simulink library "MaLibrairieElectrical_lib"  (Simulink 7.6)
settings: Solver=ode45  StartTime=0.0  StopTime=10.0  RelTol=1e-3
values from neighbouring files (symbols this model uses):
  A = [1+j -(1-j);1 -2/(1-j)]    [systeme_AX_B_phaseurs.m]
  K = 0.0005    [parametres.m]
undefined symbols (not defined in the file or in its folder): capa_reelle, F, gcbh, gen_sin_amorti, H, i, MaLibrairieElectrical, nesl_callback, Ohm, op_amp_reel, R_NL, R_NL2, rad, s, thermistance, V, v

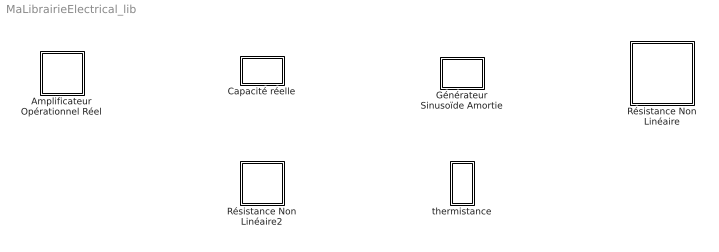
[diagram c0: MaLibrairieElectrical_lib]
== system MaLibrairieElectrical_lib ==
  Amplificateur Opérationnel Réel : Subsystem  DialogController=NetworkEngine.DynNeDlgSource  LoadFcn=nesl_callback('LoadFcn',gcbh);  mask(Amplificateur
Opérationnel Réel){ComponentPath=MaLibrairieElectrical.op_amp_reel, ClassName=op_amp_reel, SchemaVersion=1, A=1e+6, A_unit=1, Re=1e+6, Re_unit=Ohm, Rs=100, Rs_unit=Ohm, Vsat=15, Vsat_unit=V, ie_Log=off, eps_Log=off, is_Log=off, vs_Log=off, LocalVarNames=\, LocalVarDescs=ie\, LocalVarLogging=eps\}
      mask prompts: A "Gain de l'Aop en boucle ouverte"; Re "Résistance d'entrée"; Rs "Résistance de sortie"; Vsat "Tension d'alimentation"
      mask help: Dans cet amplificateur, on tient compte de: - sa résistance d'entrée Re, - sa résistance de sortie Rs, - gain en boucle ouverte, - de la saturation de la sortie à +/-Vsat
      mask init:
      | nesl_preinitmask (gcb);
  Capacité réelle : Subsystem  DialogController=NetworkEngine.DynNeDlgSource  LoadFcn=nesl_callback('LoadFcn',gcbh);  mask(Capacité réelle){ComponentPath=MaLibrairieElectrical.capa_reelle, ClassName=capa_reelle, SchemaVersion=1, C=1e-6, C_unit=F, v0=0, v0_unit=V, Rs=1e-6, Rs_unit=Ohm, Rp=1e+6, Rp_unit=Ohm, Ls=0, Ls_unit=H, vc_Log=off, v_Log=off, i_Log=off, LocalVarNames=\, LocalVarDescs=vc\, LocalVarLogging=v\}
      mask prompts: C "Capacité"; v0 "charge initiale de la capacité"; Rs "Résistance série Rs"; Rp "Résistance parallèle Rp"; Ls "Inductance série Ls"
      mask help: Cette capacité est composée d'une capacité idéale en parallèle à une résistance Rp le tout en série à une résistance Rs et une inductance Ls
      mask init:
      | nesl_preinitmask (gcb);
  Générateur Sinusoïde Amortie : Subsystem  DialogController=NetworkEngine.DynNeDlgSource  LoadFcn=nesl_callback('LoadFcn',gcbh);  mask(Générateur Sinusoïde
Amortie){ComponentPath=MaLibrairieElectrical.gen_sin_amorti, ClassName=gen_sin_amorti, SchemaVersion=1, biais=0, biais_unit=1, w=6.2832, w_unit=1/s, Amp=1, Amp_unit=1, phi=6.2832, phi_unit=rad, a=5, a_unit=1, LocalVarNames=, LocalVarDescs=, LocalVarLogging=[]}
      mask prompts: w "pulsation"; Amp "Amplitude"; phi "Phase"; a "décrément"
      mask help: Ce bloc génère le signal suivant x(t)=Amp exp(-at) sin (wt+phi)+ biais
      mask init:
      | nesl_preinitmask (gcb);
  Résistance Non Linéaire : Subsystem  DialogController=NetworkEngine.DynNeDlgSource  LoadFcn=nesl_callback('LoadFcn',gcbh);  mask(Résistance Non
Linéaire){ComponentPath=MaLibrairieElectrical.R_NL, ClassName=R_NL, SchemaVersion=1, K=10, K_unit=V/A^2, v_Log=off, i_Log=off, LocalVarNames=\, LocalVarDescs=v\, LocalVarLogging=i}
      mask prompts: K "Coefficient de la Résistance non linéaire"
      mask help: Ce composant définit une résistance non linéaire La valeur de la résistance dépend du courant qui la traverse La caractéristique est donnée par la relation entre le courant qui traverse la résistance et la tension à ses bornes U=K*i^2
      mask init:
      | nesl_preinitmask (gcb);
  Résistance Non Linéaire2 : Subsystem  DialogController=NetworkEngine.DynNeDlgSource  LoadFcn=nesl_callback('LoadFcn',gcbh);  mask(Résistance Non
Linéaire2){ComponentPath=MaLibrairieElectrical.R_NL2, ClassName=R_NL2, SchemaVersion=1, R0=10, R0_unit=Ohm, K=10, K_unit=V/A^2, i_Log=off, v_Log=off, LocalVarNames=\, LocalVarDescs=i\, LocalVarLogging=v}
      mask prompts: K "Coefficient de la Résistance non linéaire"
      mask help: Ce composant définit une résistance non linéaire La valeur de la résistance dépend du courant qui la traverse La caractéristique est donnée par la relation entre le courant qui traverse la résistance et la tension à ses bornes U=K*i^2
      mask init:
      | nesl_preinitmask (gcb);
  thermistance : Subsystem  DialogController=NetworkEngine.DynNeDlgSource  LoadFcn=nesl_callback('LoadFcn',gcbh);  mask(thermistance){ComponentPath=MaLibrairieElectrical.thermistance, ClassName=thermistance, SchemaVersion=1, T0=300, T0_unit=K, B=2.9e+3, B_unit=K, R0=100, R0_unit=Ohm, LocalVarNames=, LocalVarDescs=, LocalVarLogging=[]}
      mask prompts: T0 "Température nominale"; B "sensibilité thermique"; R0 "résistance nominale en Ohms"
      mask help: Ce composant définit un capteur de température à coefficient de température négatif La valeur de la résistance de ce capteur est donné par l'expression suivante: R(T)=R(T0) exp(B(1/T - 1/T0)) avec T et T0 en °K
      mask init:
      | nesl_preinitmask (gcb);

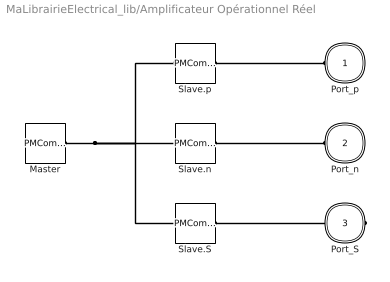
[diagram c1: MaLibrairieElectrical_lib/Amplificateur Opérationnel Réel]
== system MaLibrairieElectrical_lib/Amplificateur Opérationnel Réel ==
  Master : PMComponent  Tag=MaLibrairieElectrical.op_amp_reel  PhysicalDomain=network_engine_domain  SubClassName=master  LeftPortType=generic  RightPortType=generic  RConnTagsString=RConn1
  Slave.S : PMComponent  Tag=S  PhysicalDomain=network_engine_domain  SubClassName=terminal  LeftPortType=generic  RightPortType=foundation.electrical.electrical  LConnTagsString=LConn1  RConnTagsString=RConn1
  Slave.n : PMComponent  Tag=n  PhysicalDomain=network_engine_domain  SubClassName=terminal  LeftPortType=generic  RightPortType=foundation.electrical.electrical  LConnTagsString=LConn1  RConnTagsString=RConn1
  Slave.p : PMComponent  Tag=p  PhysicalDomain=network_engine_domain  SubClassName=terminal  LeftPortType=generic  RightPortType=foundation.electrical.electrical  LConnTagsString=LConn1  RConnTagsString=RConn1
  Port_p : PMIOPort  Tag=p  Port=1  Side=Left
  Port_n : PMIOPort  Tag=n  Port=2  Side=Left
  Port_S : PMIOPort  Tag=S  Port=3  Side=Right
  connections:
  Slave.p/RConn1 -- Port_p/RConn1
  Slave.p/LConn1 -- Slave.n/LConn1 -- Master/RConn1 -- Slave.S/LConn1
  Slave.n/RConn1 -- Port_n/RConn1
  Slave.S/RConn1 -- Port_S/RConn1

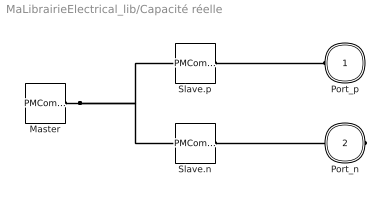
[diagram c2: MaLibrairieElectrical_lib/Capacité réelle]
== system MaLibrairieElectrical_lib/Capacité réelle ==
  Master : PMComponent  Tag=MaLibrairieElectrical.capa_reelle  PhysicalDomain=network_engine_domain  SubClassName=master  LeftPortType=generic  RightPortType=generic  RConnTagsString=RConn1
  Slave.n : PMComponent  Tag=n  PhysicalDomain=network_engine_domain  SubClassName=terminal  LeftPortType=generic  RightPortType=foundation.electrical.electrical  LConnTagsString=LConn1  RConnTagsString=RConn1
  Slave.p : PMComponent  Tag=p  PhysicalDomain=network_engine_domain  SubClassName=terminal  LeftPortType=generic  RightPortType=foundation.electrical.electrical  LConnTagsString=LConn1  RConnTagsString=RConn1
  Port_p : PMIOPort  Tag=p  Port=1  Side=Left
  Port_n : PMIOPort  Tag=n  Port=2  Side=Right
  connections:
  Slave.p/RConn1 -- Port_p/RConn1
  Master/RConn1 -- Slave.p/LConn1 -- Slave.n/LConn1
  Slave.n/RConn1 -- Port_n/RConn1

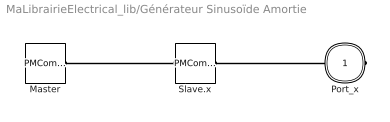
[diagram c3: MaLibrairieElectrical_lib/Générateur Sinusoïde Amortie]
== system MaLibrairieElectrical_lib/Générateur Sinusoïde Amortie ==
  Master : PMComponent  Tag=MaLibrairieElectrical.gen_sin_amorti  PhysicalDomain=network_engine_domain  SubClassName=master  LeftPortType=generic  RightPortType=generic  RConnTagsString=RConn1
  Slave.x : PMComponent  Tag=x  PhysicalDomain=network_engine_domain  SubClassName=output  LeftPortType=generic  RightPortType=output  LConnTagsString=LConn1  RConnTagsString=RConn1
  Port_x : PMIOPort  Tag=x  Port=1  Side=Right
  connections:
  Slave.x/RConn1 -- Port_x/RConn1
  Slave.x/LConn1 -- Master/RConn1

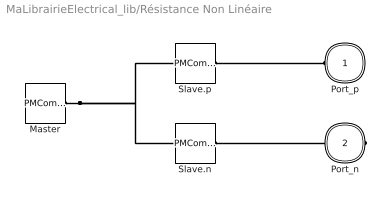
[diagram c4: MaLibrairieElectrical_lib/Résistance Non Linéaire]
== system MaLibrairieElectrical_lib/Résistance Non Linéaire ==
  Master : PMComponent  Tag=MaLibrairieElectrical.R_NL  PhysicalDomain=network_engine_domain  SubClassName=master  LeftPortType=generic  RightPortType=generic  RConnTagsString=RConn1
  Slave.n : PMComponent  Tag=n  PhysicalDomain=network_engine_domain  SubClassName=terminal  LeftPortType=generic  RightPortType=foundation.electrical.electrical  LConnTagsString=LConn1  RConnTagsString=RConn1
  Slave.p : PMComponent  Tag=p  PhysicalDomain=network_engine_domain  SubClassName=terminal  LeftPortType=generic  RightPortType=foundation.electrical.electrical  LConnTagsString=LConn1  RConnTagsString=RConn1
  Port_p : PMIOPort  Tag=p  Port=1  Side=Left
  Port_n : PMIOPort  Tag=n  Port=2  Side=Right
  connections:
  Slave.p/RConn1 -- Port_p/RConn1
  Master/RConn1 -- Slave.p/LConn1 -- Slave.n/LConn1
  Slave.n/RConn1 -- Port_n/RConn1

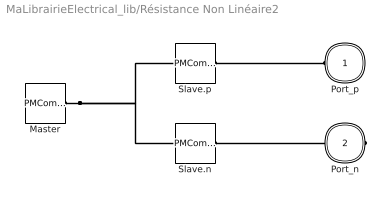
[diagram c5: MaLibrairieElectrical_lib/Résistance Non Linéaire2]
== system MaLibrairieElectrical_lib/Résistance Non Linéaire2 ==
  Master : PMComponent  Tag=MaLibrairieElectrical.R_NL2  PhysicalDomain=network_engine_domain  SubClassName=master  LeftPortType=generic  RightPortType=generic  RConnTagsString=RConn1
  Slave.n : PMComponent  Tag=n  PhysicalDomain=network_engine_domain  SubClassName=terminal  LeftPortType=generic  RightPortType=foundation.electrical.electrical  LConnTagsString=LConn1  RConnTagsString=RConn1
  Slave.p : PMComponent  Tag=p  PhysicalDomain=network_engine_domain  SubClassName=terminal  LeftPortType=generic  RightPortType=foundation.electrical.electrical  LConnTagsString=LConn1  RConnTagsString=RConn1
  Port_p : PMIOPort  Tag=p  Port=1  Side=Left
  Port_n : PMIOPort  Tag=n  Port=2  Side=Right
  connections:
  Slave.p/RConn1 -- Port_p/RConn1
  Master/RConn1 -- Slave.p/LConn1 -- Slave.n/LConn1
  Slave.n/RConn1 -- Port_n/RConn1

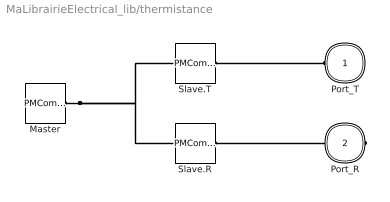
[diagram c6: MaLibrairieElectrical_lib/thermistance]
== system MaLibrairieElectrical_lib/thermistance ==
  Master : PMComponent  Tag=MaLibrairieElectrical.thermistance  PhysicalDomain=network_engine_domain  SubClassName=master  LeftPortType=generic  RightPortType=generic  RConnTagsString=RConn1
  Slave.R : PMComponent  Tag=R  PhysicalDomain=network_engine_domain  SubClassName=output  LeftPortType=generic  RightPortType=output  LConnTagsString=LConn1  RConnTagsString=RConn1
  Slave.T : PMComponent  Tag=T  PhysicalDomain=network_engine_domain  SubClassName=input  LeftPortType=generic  RightPortType=input  LConnTagsString=LConn1  RConnTagsString=RConn1
  Port_T : PMIOPort  Tag=T  Port=1  Side=Left
  Port_R : PMIOPort  Tag=R  Port=2  Side=Right
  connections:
  Slave.T/RConn1 -- Port_T/RConn1
  Master/RConn1 -- Slave.T/LConn1 -- Slave.R/LConn1
  Slave.R/RConn1 -- Port_R/RConn1
